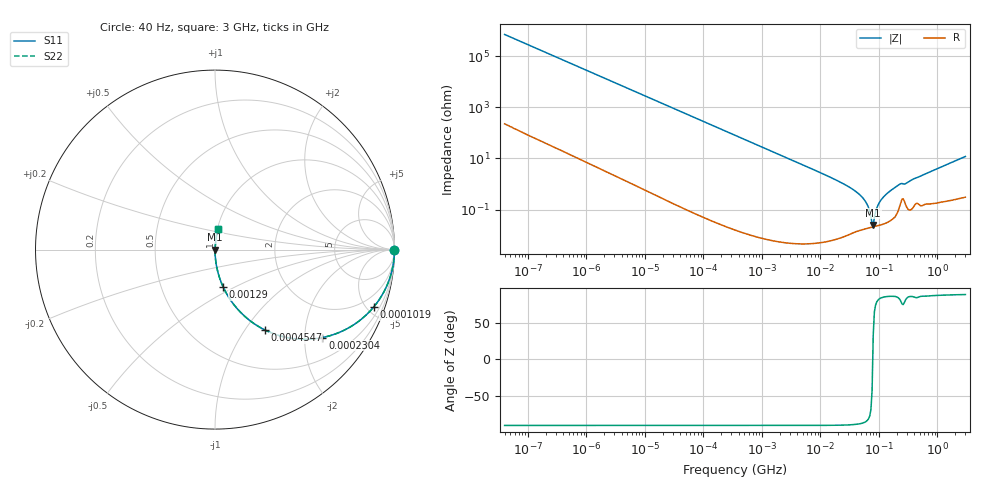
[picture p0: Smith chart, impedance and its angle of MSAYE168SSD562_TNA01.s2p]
! MSAYE168SSD562_TNA01  S-PARAMETER MODEL  ( General Type )
! Model Generated by TAIYO YUDEN Corporation (http://www.ty-top.com)
! Version 2.0
! TAIYO YUDEN Control No. 031107
! Copyright(c) 2003 TAIYO YUDEN CO.,LTD. All Rights Reserved.
! Product Description (link to TY-COMPAS)
! https://ds.yuden.co.jp/TYCOMPAS/or/detail?pn=MSAYE168SSD562KTNA01&u=M
! Products Name : Multilayer Ceramic Capacitors
! Characteristics :
!  Capacitance : 5600 pF , Rated Voltage : 16V
!  Case Size : 1.6 x 0.8 / 0.063 x 0.031 [mm/inch] , Thickness : 0.8 / 0.031 [mm/inch]
!  (Conditions: Temperature = 25 degC , DC Bias Current/Voltage = 0A / 0V)
! External Node Assignments :
!  1  o---| |---o  2
! GND o---------o GND
! Frequency Range : 40Hz  -  3GHz  [ 401 STEP ]
# MHz S RI R 50
! Freq[MHz].  S11 Real  S11 Imag  S21 Real  S21 Imag  S12 Real  S12 Imag  S22 Real  S22 Imag
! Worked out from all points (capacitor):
!   401 points, 40 Hz to 3 GHz, reference 50 ohm
!   read as one part in series: C = 5.66 nF near 44 Hz
!   lowest |Z| = 25.2 mohm at 79.82 MHz (marker M1)
!   series resonance near 78.31 MHz, so ESL is about 730 pH
!   S11 on the Smith chart (normalised r, x): 40 Hz: open; 101.9 kHz: 1.00, -5.52; 230.4 kHz: 1.00, -2.44; 454.7 kHz: 1.00, -1.24; 1.29 MHz: 1.00, -0.44; 3 GHz: 1.01, +0.24
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4e-05  1 -0.000142  6.6e-08 0.000142  6.6e-08 0.000142  1 -0.000142
0.000834  1 -0.00297  9.57e-06 0.00297  9.57e-06 0.00297  1 -0.00297
0.017386  0.9962 -0.0616  0.00383 0.0616  0.00383 0.0616  0.9962 -0.0616
0.101865  0.8838 -0.3204  0.1162 0.3204  0.1162 0.3204  0.8838 -0.3204
0.230357  0.5981 -0.4902  0.4019 0.4902  0.4019 0.4902  0.5981 -0.4902
0.362475  0.3754 -0.4841  0.6246 0.4841  0.6246 0.4841  0.3754 -0.4841
0.454691  0.2764 -0.4471  0.7236 0.4471  0.7236 0.4471  0.2764 -0.4471
1.28983  0.0453 -0.2079  0.9547 0.2079  0.9547 0.2079  0.0453 -0.2079
7.222098  0.00153 -0.0385  0.9985 0.0385  0.9985 0.0385  0.00153 -0.0385
22.43131  0.00021 -0.0115  0.9998 0.0115  0.9998 0.0115  0.00021 -0.0115
42.31378  0.000163 -0.00466  0.9998 0.00466  0.9998 0.00466  0.000163 -0.00466
58.11596  0.00018 -0.00216  0.9998 0.00216  0.9998 0.00216  0.00018 -0.00216
66.58224  0.000192 -0.00116  0.9998 0.00116  0.9998 0.00116  0.000192 -0.00116
72.90103  0.000201 -0.000503  0.9998 0.000503  0.9998 0.000503  0.000201 -0.000503
79.8195  0.000211 0.000138  0.9998 -0.000138  0.9998 -0.000138  0.000211 0.000138
83.52119  0.000216 0.000462  0.9998 -0.000462  0.9998 -0.000462  0.000216 0.000462
95.68847  0.000235 0.00143  0.9998 -0.00143  0.9998 -0.00143  0.000235 0.00143
104.7695  0.000251 0.0021  0.9997 -0.0021  0.9997 -0.0021  0.000251 0.0021
150.5692  0.000372 0.00506  0.9996 -0.00506  0.9996 -0.00506  0.000372 0.00506
226.4253  0.00146 0.00969  0.9985 -0.00969  0.9985 -0.00969  0.00146 0.00969
297.2015  0.00137 0.0108  0.9986 -0.0108  0.9986 -0.0108  0.00137 0.0108
3000  0.0169 0.1169  0.9831 -0.1169  0.9831 -0.1169  0.0169 0.1169
